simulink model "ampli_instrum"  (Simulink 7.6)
settings: Solver=ode15s  StartTime=0.0  StopTime=0.004  RelTol=1e-3
StopFcn:
  | close all, clc
  | load signaux_es.mat
  | plot(x(1,:),x(2,:),x(1,:),x(3,:),x(1,:),x(4,:))
  | title('Amplificateur d''instrumentation')
  | xlabel('temps')
  | grid
libraries: fl_lib x14, nesl_utility x4, simulink x1

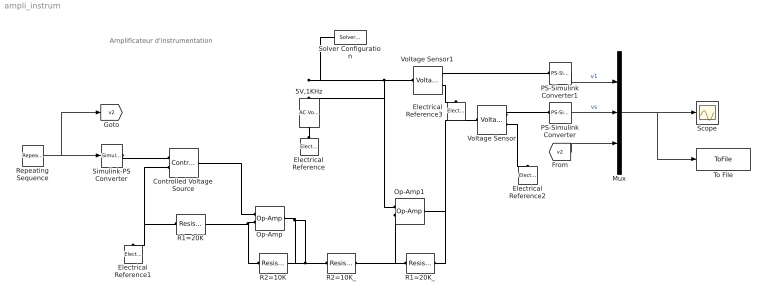
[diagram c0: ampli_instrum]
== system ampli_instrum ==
  note: Amplificateur d'instrumentation
  5V,1KHz : fl_lib/Electrical/Electrical Sources/AC Voltage Source  DialogController=NetworkEngine.DynNeDlgSource  SystemSampleTime=-1  amp=2 V  shift=0 rad  omega=1000 Hz  i_Log=off  v_Log=off  LocalVarNames=|current|voltage|power  LocalVarDescs=|Current (A)|Voltage (V)|Power (W)  LocalVarLogging=[0 0 0]
  Controlled Voltage Source : fl_lib/Electrical/Electrical Sources/Controlled Voltage Source  DialogController=NetworkEngine.DynNeDlgSource  SystemSampleTime=-1  i_Log=off  v_Log=off  LocalVarNames=|i|v  LocalVarDescs=|i|v  LocalVarLogging=[0 0]
  Electrical Reference{,1..3} (4 alike) : fl_lib/Electrical/Electrical Elements/Electrical Reference  DialogController=NetworkEngine.DynNeDlgSource  SystemSampleTime=-1  i_Log=off  LocalVarNames=|i  LocalVarDescs=|i  LocalVarLogging=[]
  Mux : Mux  Inputs=3
  Op-Amp : fl_lib/Electrical/Electrical Elements/Op-Amp  DialogController=NetworkEngine.DynNeDlgSource  SystemSampleTime=-1  i1_Log=off  v1_Log=off  outI_Log=off  LocalVarNames=|i1|v1|outI  LocalVarDescs=|i1|v1|outI  LocalVarLogging=[]
  Op-Amp1 : fl_lib/Electrical/Electrical Elements/Op-Amp  DialogController=NetworkEngine.DynNeDlgSource  SystemSampleTime=-1  i1_Log=off  v1_Log=off  outI_Log=off  LocalVarNames=|i1|v1|outI  LocalVarDescs=|i1|v1|outI  LocalVarLogging=[]
  PS-Simulink Converter : nesl_utility/PS-Simulink Converter  DialogController=NetworkEngine.DynNeUtilDlgSource  SystemSampleTime=-1  PhysicalDomain=network_engine_domain  LeftPortType=input  RightPortType=output  SubClassName=ps_output  Unit=1  AffineConversion=off
  PS-Simulink Converter1 : nesl_utility/PS-Simulink Converter  DialogController=NetworkEngine.DynNeUtilDlgSource  SystemSampleTime=-1  PhysicalDomain=network_engine_domain  LeftPortType=input  RightPortType=output  SubClassName=ps_output  Unit=1  AffineConversion=off
  R1=20K : fl_lib/Electrical/Electrical Elements/Resistor  DialogController=NetworkEngine.DynNeDlgSource  SystemSampleTime=-1  R=20 kOhm  i_Log=off  v_Log=off  LocalVarNames=|current|voltage|power  LocalVarDescs=|Resistor current (A)|Voltage across resistor (V)|Power (W)  LocalVarLogging=[0 0 0]
  R1=20K_ : fl_lib/Electrical/Electrical Elements/Resistor  DialogController=NetworkEngine.DynNeDlgSource  SystemSampleTime=-1  R=20e3 Ohm  i_Log=off  v_Log=off  LocalVarNames=|current|voltage|power  LocalVarDescs=|Resistor current (A)|Voltage across resistor (V)|Power (W)  LocalVarLogging=[0 0 0]
  R2=10K : fl_lib/Electrical/Electrical Elements/Resistor  DialogController=NetworkEngine.DynNeDlgSource  SystemSampleTime=-1  R=10 kOhm  i_Log=off  v_Log=off  LocalVarNames=|current|voltage|power  LocalVarDescs=|Resistor current (A)|Voltage across resistor (V)|Power (W)  LocalVarLogging=[0 0 0]
  R2=10K_ : fl_lib/Electrical/Electrical Elements/Resistor  DialogController=NetworkEngine.DynNeDlgSource  SystemSampleTime=-1  R=10e3 Ohm  i_Log=off  v_Log=off  LocalVarNames=|current|voltage|power  LocalVarDescs=|Resistor current (A)|Voltage across resistor (V)|Power (W)  LocalVarLogging=[0 0 0]
  Repeating Sequence : simulink/Sources/Repeating Sequence  SystemSampleTime=-1  rep_seq_t=[0 0.001 0.002]  rep_seq_y=[0 1 0]
  Scope : Scope
  Simulink-PS Converter : nesl_utility/Simulink-PS Converter  DialogController=NetworkEngine.DynNeUtilDlgSource  SystemSampleTime=-1  PhysicalDomain=network_engine_domain  LeftPortType=input  RightPortType=output  SubClassName=ps_input  Unit=1  AffineConversion=off  InputFilterTimeConstant=.001  UdotUserProvided=0
  Solver Configuration : nesl_utility/Solver Configuration  DialogController=NetworkEngine.DynNeUtilDlgSource  SystemSampleTime=-1  PhysicalDomain=network_engine_domain  LeftPortType=input  RightPortType=generic  SubClassName=solver  Accelerate=off  Profile=off  ResidualTolerance=1e-9  MaxNonlinIter=12  MaxModeIter=2  DoFixedCost=off  UseLocalSampling=off  DoDC=off  LinearAlgebra=Sparse  LocalSolverSampleTime=.001  LocalSolverChoice=NE_BACKWARD_EULER_ADVANCER  UseLocalSolver=off
  To File : ToFile  Filename=signaux_es  MatrixName=x
  Voltage Sensor : fl_lib/Electrical/Electrical Sensors/Voltage Sensor  DialogController=NetworkEngine.DynNeDlgSource  SystemSampleTime=-1  i1_Log=off  v1_Log=off  LocalVarNames=|i1|v1  LocalVarDescs=|i1|v1  LocalVarLogging=[]
  Voltage Sensor1 : fl_lib/Electrical/Electrical Sensors/Voltage Sensor  DialogController=NetworkEngine.DynNeDlgSource  SystemSampleTime=-1  i1_Log=off  v1_Log=off  LocalVarNames=|i1|v1  LocalVarDescs=|i1|v1  LocalVarLogging=[]
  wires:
  PS-Simulink Converter1/1 -> Mux/1  "v1"
  PS-Simulink Converter/1 -> Mux/2  "vs"
  Mux/1 -> Scope/1, To File/1
  Repeating Sequence/1 -> Simulink-PS Converter/1, [v2]
  [v2] -> Mux/3
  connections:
  R1=20K/LConn1 -- Controlled Voltage Source/RConn2 -- Electrical Reference1/LConn1
  R2=10K/LConn1 -- Op-Amp/LConn2 -- R1=20K/RConn1
  Op-Amp/RConn1 -- R2=10K/RConn1 -- R2=10K_/LConn1
  R1=20K_/LConn1 -- R2=10K_/RConn1 -- Op-Amp1/LConn2
  Voltage Sensor/RConn1 -- PS-Simulink Converter/LConn1
  Voltage Sensor/RConn2 -- Electrical Reference2/LConn1
  Voltage Sensor1/RConn1 -- PS-Simulink Converter1/LConn1
  Voltage Sensor1/RConn2 -- Electrical Reference3/LConn1
  5V,1KHz/RConn1 -- Electrical Reference/LConn1
  R1=20K_/RConn1 -- Op-Amp1/RConn1 -- Voltage Sensor/LConn1
  Solver Configuration/RConn1 -- 5V,1KHz/LConn1 -- Op-Amp1/LConn1 -- Voltage Sensor1/LConn1
  Simulink-PS Converter/RConn1 -- Controlled Voltage Source/RConn1
  Op-Amp/LConn1 -- Controlled Voltage Source/LConn1
